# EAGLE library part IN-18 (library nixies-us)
IN-18: large numeric frontview nixie tube
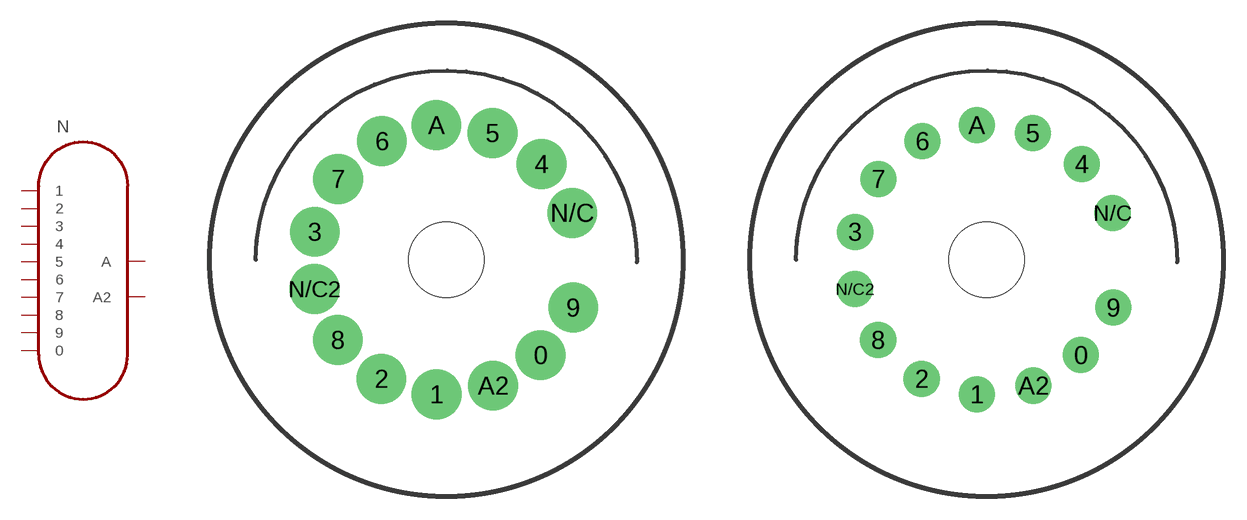
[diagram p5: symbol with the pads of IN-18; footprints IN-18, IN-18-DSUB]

Designator prefix N

## IN-18  [IN-18]
0  0
1  1
2  2
3  3
4  4
5  5
6  6
7  7
8  8
9  9
A  A
A2  A2

## IN-18D-SUB  [IN-18-DSUB]
Pads as for IN-18

## IN-18MILL-MAX  [IN-18-8331]
Pads as for IN-18

## Footprint IN-18 (pad centres in mm)
May be used with socket: PL31-P
drill 2.3 pad 3.2: 0 6.282,-6.357; 1 -0.645,-8.971; 2 -4.33,-7.938; 3 -8.76,1.863; 4 6.35,6.382; 5 3.09,8.449; 6 -4.291,7.907; 7 -7.214,5.386; 8 -7.228,-5.344; 9 8.456,-3.189; A -0.659,8.976; A2 3.123,-8.394; N/C 8.394,3.123; N/C2 -8.781,-1.948
hole 5 at 0,0

## Footprint IN-18-DSUB (pad centres in mm)
May be used with socket: PL31-P
drill 1.6: 0 6.282,-6.357; 1 -0.645,-8.971; 2 -4.33,-7.938; 3 -8.76,1.863; 4 6.35,6.382; 5 3.09,8.449; 6 -4.291,7.907; 7 -7.214,5.386; 8 -7.228,-5.344; 9 8.456,-3.189; A -0.659,8.976; A2 3.123,-8.394; N/C 8.394,3.123; N/C2 -8.781,-1.948
hole 5 at 0,0

## Footprint IN-18-8331 (pad centres in mm)
May be used with socket: PL31-P
drill 1.829: 0 6.282,-6.357; 1 -0.645,-8.971; 2 -4.33,-7.938; 3 -8.76,1.863; 4 6.35,6.382; 5 3.09,8.449; 6 -4.291,7.907; 7 -7.214,5.386; 8 -7.228,-5.344; 9 8.456,-3.189; A -0.659,8.976; A2 3.123,-8.394; N/C 8.394,3.123; N/C2 -8.781,-1.948
hole 5 at 0,0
